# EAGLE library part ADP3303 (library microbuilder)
ADP3303 - High Accuracy 200 mA LDO Digikey: 3.3V - ADP3303ARZ-3.3-ND Input: 3.5-12V Vf: 180mV @ 200mA Temp: -20°C-85°C Digikey: 5.0V - ADP3303ARZ-5-ND
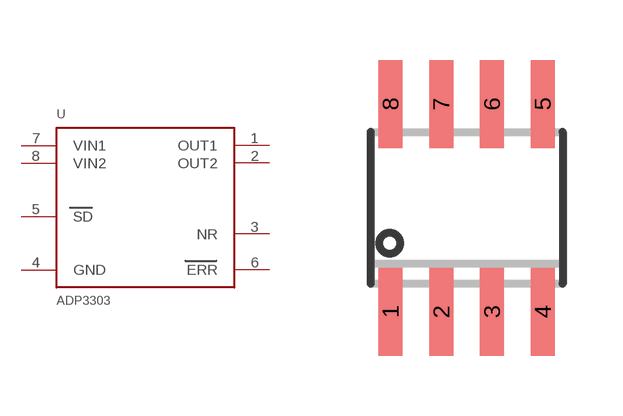
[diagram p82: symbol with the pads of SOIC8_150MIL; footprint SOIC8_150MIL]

Designator prefix U

## ADP3303  [SOIC8_150MIL]
1  OUT1
2  OUT2
3  NR
4  GND
5  SD
6  ERR
7  VIN1
8  VIN2

## Footprint SOIC8_150MIL (pad centres in mm)
Small Outline IC - 150mil Wide
smd 0.6 x 2.2: 1 -1.905,-2.6; 2 -0.635,-2.6; 3 0.635,-2.6; 4 1.905,-2.6; 5 1.905,2.6; 6 0.635,2.6; 7 -0.635,2.6; 8 -1.905,2.6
